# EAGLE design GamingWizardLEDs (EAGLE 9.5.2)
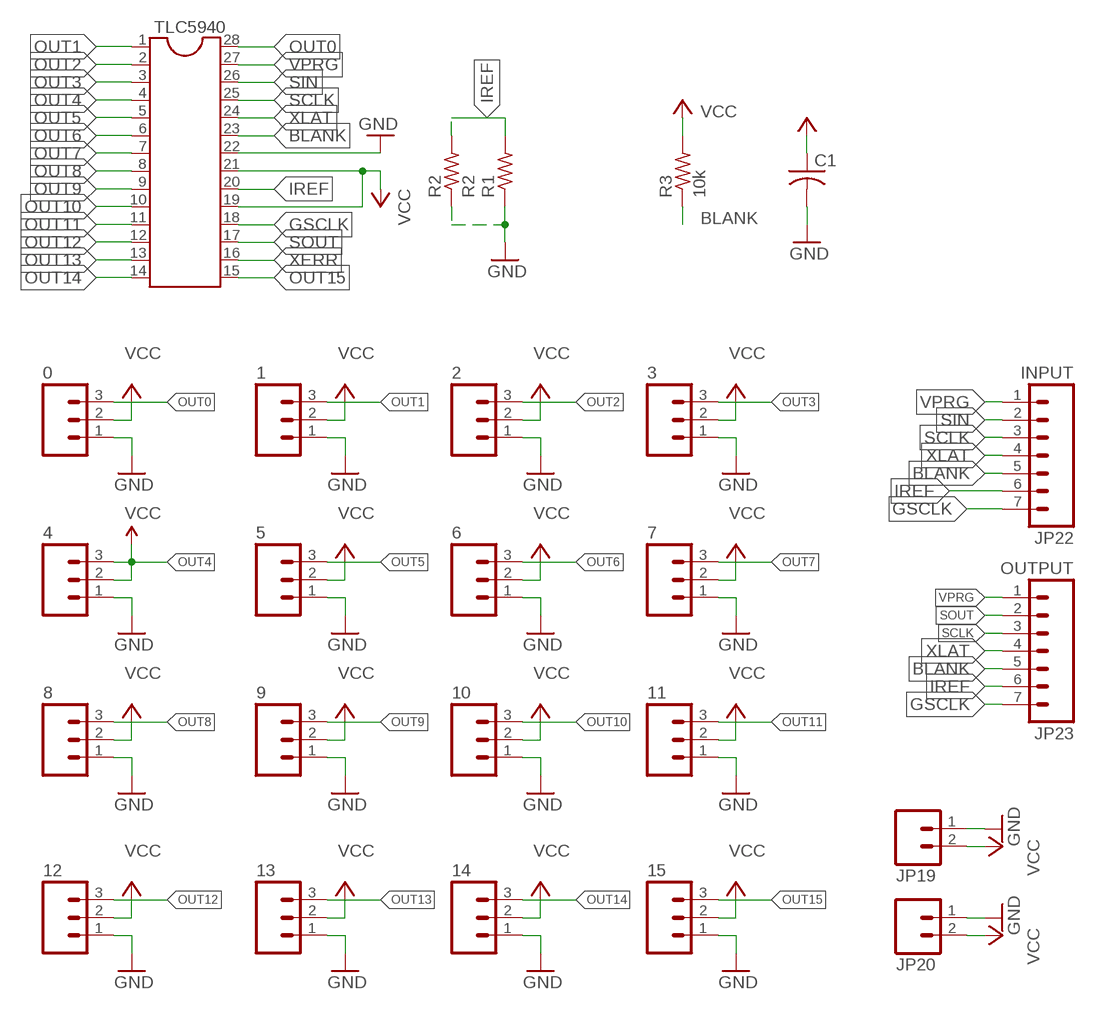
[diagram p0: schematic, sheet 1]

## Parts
0  M03PTH  [1X03]
1  M03PTH  [1X03]
2  M03PTH  [1X03]
3  M03PTH  [1X03]
4  M03PTH  [1X03]
5  M03PTH  [1X03]
6  M03PTH  [1X03]
7  M03PTH  [1X03]
8  M03PTH  [1X03]
9  M03PTH  [1X03]
10  M03PTH  [1X03]
11  M03PTH  [1X03]
12  M03PTH  [1X03]
13  M03PTH  [1X03]
14  M03PTH  [1X03]
15  M03PTH  [1X03]
C1  100nF  C-USC0805  [C0805]
JP19  M02PTH  [1X02]
JP20  M02PTH  [1X02]
JP22  INPUT  M07  [1X07]
JP23  OUTPUT  M07  [1X07]
R1  2.2k  R-US_R0805  [R0805]
R2  R2  R-US_R0805  [R0805]
R3  10k  R-US_R0805  [R0805]
TLC5940  DIL28-3  [DIL28-3]

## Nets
BLANK: JP22.5 JP23.5 R3.1 TLC5940.23
GND: 0.1 1.1 2.1 3.1 4.1 5.1 6.1 7.1 8.1 9.1 10.1 11.1 12.1 13.1 14.1 15.1 C1.2 JP19.1 JP20.1 R1.1 R2.1 TLC5940.22
GSCLK: JP22.7 JP23.7 TLC5940.18
IREF: JP22.6 JP23.6 R1.2 R2.2 TLC5940.20
OUT0: 0.3 TLC5940.28
OUT1: 1.3 TLC5940.1
OUT2: 2.3 TLC5940.2
OUT3: 3.3 TLC5940.3
OUT4: 4.3 TLC5940.4
OUT5: 5.3 TLC5940.5
OUT6: 6.3 TLC5940.6
OUT7: 7.3 TLC5940.7
OUT8: 8.3 TLC5940.8
OUT9: 9.3 TLC5940.9
OUT10: 10.3 TLC5940.10
OUT11: 11.3 TLC5940.11
OUT12: 12.3 TLC5940.12
OUT13: 13.3 TLC5940.13
OUT14: 14.3 TLC5940.14
OUT15: 15.3 TLC5940.15
SCLK: JP22.3 JP23.3 TLC5940.25
SIN: JP22.2 TLC5940.26
SOUT: JP23.2 TLC5940.17
VCC: 0.2 1.2 2.2 3.2 4.2 5.2 6.2 7.2 8.2 9.2 10.2 11.2 12.2 13.2 14.2 15.2 C1.1 JP19.2 JP20.2 R3.2 TLC5940.19 TLC5940.21
VPRG: JP22.1 JP23.1 TLC5940.27
XERR: TLC5940.16
XLAT: JP22.4 JP23.4 TLC5940.24

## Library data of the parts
0 1-15 = SparkFun:M03: Header 3 Standard 3-pin 0.1" header. Use with straight break away headers (SKU : PRT-00116), right angle break away headers (PRT-00553), swiss pins (PRT-00743), machine pins (PRT-00117), and female headers (PRT-00115). Molex polarized connector foot print use with SKU : PRT-08232 with associated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
C1 = rcl:C-US: CAPACITOR, American symbol; MANUFACTURER: Samsung Electro-Mechanics; MANUFACTURER_PART_NUMBER: CL21F104ZBCNNNC; SPICEPREFIX: C
JP19 JP20 = SparkFun:M02: Header 2
JP22 JP23 = SparkFun:M07: Header 7 Standard 7-pin 0.1" header. Use with straight break away headers (SKU : PRT-00116), right angle break away headers (PRT-00553), swiss pins (PRT-00743), machine pins (PRT-00117), and female headers (PRT-00115). NOTES ON THE VARIANTS LOCK and LOCK_LONGPADS... This footprint was designed to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
R1 = rcl:R-US_: RESISTOR, American symbol; MANUFACTURER: UNI-ROYAL(Uniroyal Elec); MANUFACTURER_PART_NUMBER: 0805W8J0222T5E; SPICEPREFIX: R
R2 = rcl:R-US_: RESISTOR, American symbol; SPICEPREFIX: R
R3 = rcl:R-US_: RESISTOR, American symbol; MANUFACTURER: UNI-ROYAL(Uniroyal Elec); MANUFACTURER_PART_NUMBER: 0805W8F1002T5E; SPICEPREFIX: R
TLC5940 = ic-package:DIL28: Dual In Line

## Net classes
0 default: width 0.508 mm

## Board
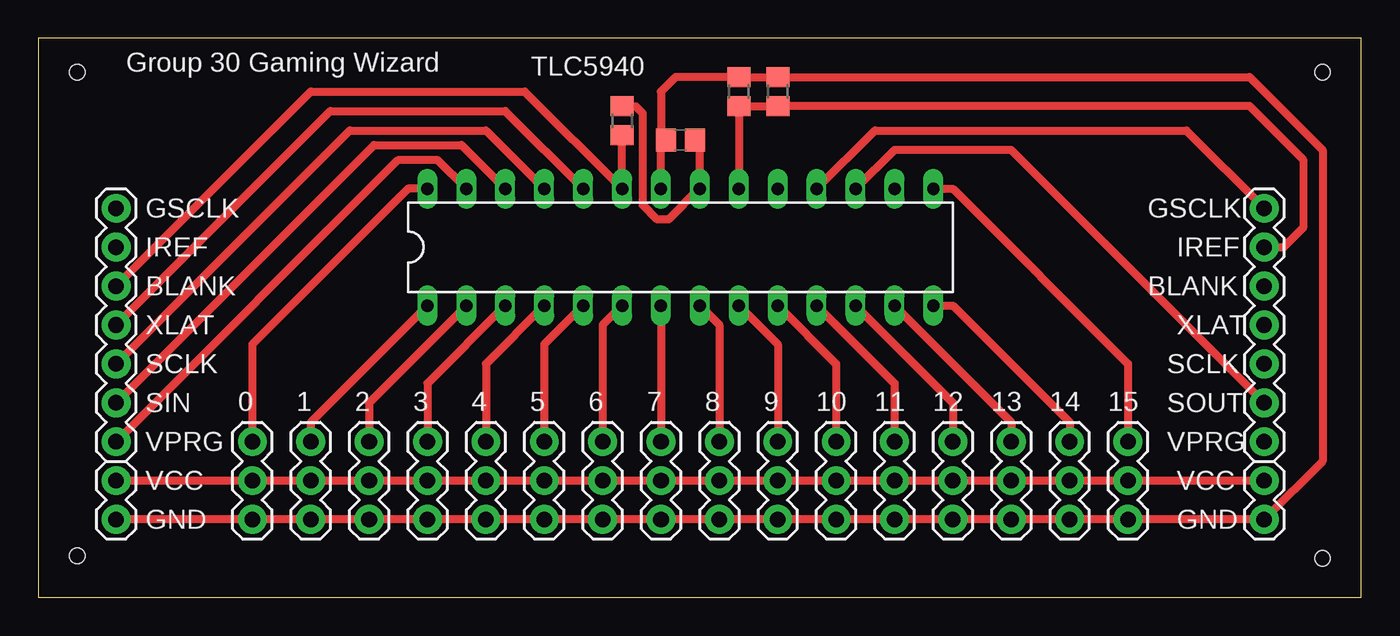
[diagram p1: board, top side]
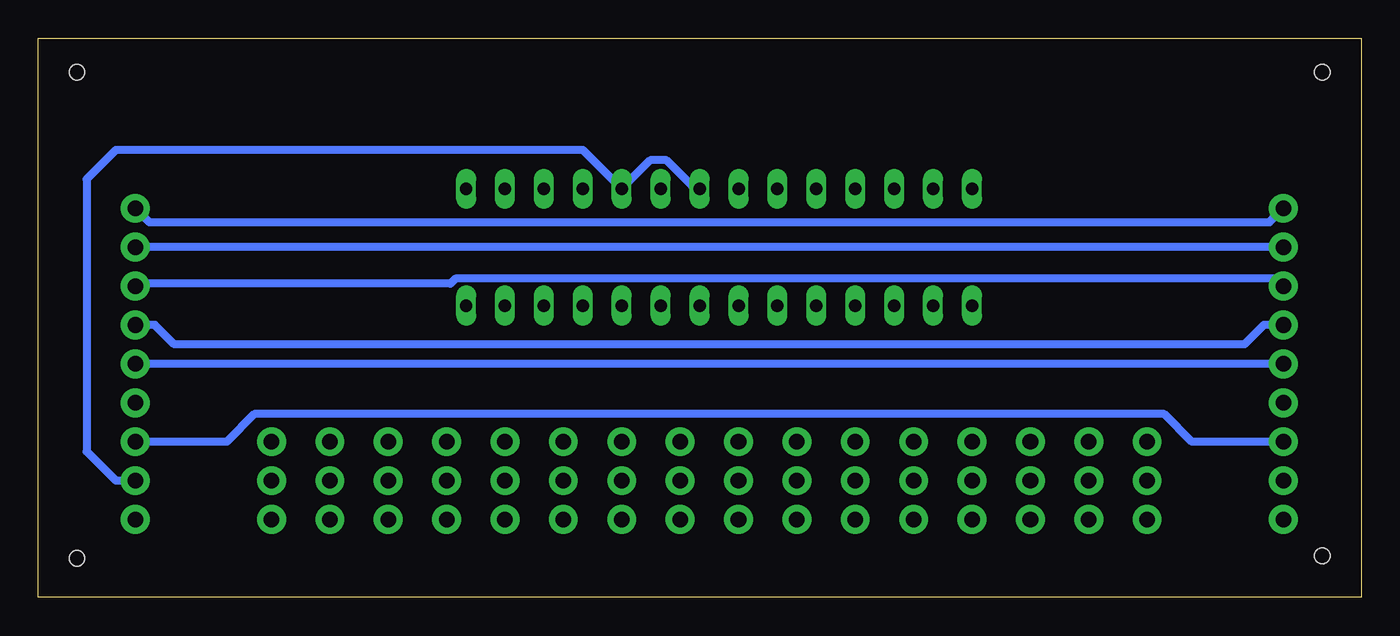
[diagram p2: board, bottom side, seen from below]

Size 86.34 x 36.5 mm. Coordinates in mm from the lower left corner, seen from the top.
Outline: 0,0 86.34,0 86.34,36.5 0,36.5 0,0
Copper layers (1*16): Top 0.035mm / dielectric 1.5mm / Bottom 0.035mm
Design rules "default": minimum track width 6mil, minimum drill 0.35mm, track to track 6mil, track to pad 6mil, pad to pad 6mil, via to via 6mil, smd to smd 6mil, copper to edge 40mil, drill to drill 6mil, minimum pad ring 10mil, minimum via ring 8mil, stop-mask expansion 4mil, vias tented up to drill 0mil, thermal gap 10mil
Holes 1 mm at 2.54,2.7 2.54,34.29 83.82,34.29 83.82,2.54

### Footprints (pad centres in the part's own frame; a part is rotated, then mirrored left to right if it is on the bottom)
1X03 = drill 1.016 pad 1.88: 1 0,0; 2 2.54,0; 3 5.08,0
C0805 = smd 1.3 x 1.5: 1 -0.95,0; 2 0.95,0
1X02 = drill 1.016 pad 1.88: 1 0,0; 2 2.54,0
1X07 = drill 1.016 pad 1.88: 1 0,0; 2 2.54,0; 3 5.08,0; 4 7.62,0; 5 10.16,0; 6 12.7,0; 7 15.24,0
R0805 = smd 1.3 x 1.5: 1 -0.95,0; 2 0.95,0
DIL28-3 = drill 0.813 long: 1 -16.51,-3.81; 2 -13.97,-3.81; 3 -11.43,-3.81; 4 -8.89,-3.81; 5 -6.35,-3.81; 6 -3.81,-3.81; 7 -1.27,-3.81; 8 1.27,-3.81; 9 3.81,-3.81; 10 6.35,-3.81; 11 8.89,-3.81; 12 11.43,-3.81; 13 13.97,-3.81; 14 16.51,-3.81; 15 16.51,3.81; 16 13.97,3.81; 17 11.43,3.81; 18 8.89,3.81; 19 6.35,3.81; 20 3.81,3.81; 21 1.27,3.81; 22 -1.27,3.81; 23 -3.81,3.81; 24 -6.35,3.81; 25 -8.89,3.81; 26 -11.43,3.81; 27 -13.97,3.81; 28 -16.51,3.81

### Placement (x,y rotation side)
0  13.97,5.08 90 top
1  17.78,5.08 90 top
2  21.59,5.08 90 top
3  25.4,5.08 90 top
4  29.21,5.08 90 top
5  33.02,5.08 90 top
6  36.83,5.08 90 top
7  40.64,5.08 90 top
8  44.45,5.08 90 top
9  48.26,5.08 90 top
10  52.07,5.08 90 top
11  55.88,5.08 90 top
12  59.69,5.08 90 top
13  63.5,5.08 90 top
14  67.31,5.08 90 top
15  71.12,5.08 90 top
C1  41.91,29.84 180 top
JP19  5.08,5.08 90 top
JP20  80.01,5.08 90 top
JP22  5.08,10.16 90 top
JP23  80.01,10.16 90 top
R1  45.72,33.02 270 top
R2  48.26,33.02 270 top
R3  38.1,31.11 90 top
TLC5940  41.91,22.86 0 top

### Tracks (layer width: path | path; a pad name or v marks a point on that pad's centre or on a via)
BLANK
  Top 0.508: JP22.5 17.78,33.02 31.75,33.02 TLC5940.23 R3.1
  Bottom 0.508: JP22.5 5.28,20.47 5.61,20.8 59.11,20.8 59.44,20.47 79.91,20.47 JP23.5
GND
  Top 0.508: JP19.1 0.1 1.1 2.1 3.1 4.1 5.1 6.1 7.1 8.1 9.1 10.1 11.1 12.1 13.1 14.1 15.1 JP20.1 83.82,8.89 83.82,29.21 79.06,33.97 R2.1 R1.1 41.59,33.97 40.64,33.02 40.64,29.84 40.8,29.68 | TLC5940.22 40.64,29.52 40.8,29.68 | 40.8,29.68 C1.2
GSCLK
  Top 0.508: TLC5940.18 54.61,30.48 74.93,30.48 JP23.7
  Bottom 0.508: JP22.7 5.99,24.49 79.1,24.49 JP23.7
IREF
  Top 0.508: TLC5940.20 R1.2 R2.2 79.06,32.07 82.55,28.57 82.55,24.13 81.28,22.86 JP23.6
  Bottom 0.508: JP22.6 JP23.6
OUT0
  Top 0.508: TLC5940.28 24.13,26.67 13.97,16.51 0.3
OUT1
  Top 0.508: TLC5940.1 17.78,11.43 1.3
OUT2
  Top 0.508: TLC5940.2 21.59,12.7 2.3
OUT3
  Top 0.508: TLC5940.3 25.4,13.97 3.3
OUT4
  Top 0.508: TLC5940.4 29.21,15.24 4.3
OUT5
  Top 0.508: TLC5940.5 33.02,16.51 5.3
OUT6
  Top 0.508: TLC5940.6 36.83,17.78 6.3
OUT7
  Top 0.508: TLC5940.7 7.3
OUT8
  Top 0.508: TLC5940.8 44.45,17.78 8.3
OUT9
  Top 0.508: TLC5940.9 48.26,16.51 9.3
OUT10
  Top 0.508: TLC5940.10 52.07,15.24 10.3
OUT11
  Top 0.508: TLC5940.11 55.88,13.97 11.3
OUT12
  Top 0.508: TLC5940.12 59.69,12.7 12.3
OUT13
  Top 0.508: TLC5940.13 63.5,11.43 13.3
OUT14
  Top 0.508: TLC5940.14 59.69,19.05 67.31,11.43 14.3
OUT15
  Top 0.508: TLC5940.15 59.69,26.67 71.12,15.24 15.3
SCLK
  Top 0.508: JP22.3 20.32,30.48 29.21,30.48 TLC5940.25
  Bottom 0.508: JP22.3 JP23.3
SIN
  Top 0.508: JP22.2 21.91,29.53 27.62,29.53 TLC5940.26
SOUT
  Top 0.508: JP23.2 63.5,29.21 55.88,29.21 TLC5940.17
VCC
  Top 0.508: JP19.2 0.2 1.2 2.2 3.2 4.2 5.2 6.2 7.2 8.2 9.2 10.2 11.2 12.2 13.2 14.2 15.2 JP20.2 | C1.1 43.18,29.52 TLC5940.21 43.13,26.67 41.13,24.68 40.39,24.68 39.47,25.6 39.47,31.59 38.99,32.06 R3.2
  Bottom 0.508: TLC5940.21 43.48,26.67 45.35,28.54 46.41,28.54 48.26,26.68 TLC5940.19 50.8,29.21 81.28,29.21 83.19,27.3 83.19,9.53 81.28,7.62 JP20.2
VPRG
  Top 0.508: JP22.1 23.46,28.54 26.07,28.54 TLC5940.27
  Bottom 0.508: JP22.1 11.05,10.16 12.85,11.96 72.24,11.96 74.04,10.16 JP23.1
XLAT
  Top 0.508: JP22.4 19.05,31.75 30.48,31.75 TLC5940.24
  Bottom 0.508: JP22.4 6.35,17.78 7.62,16.51 77.47,16.51 78.74,17.78 JP23.4

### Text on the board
tNames: Group 30 Gaming Wizard | GSCLK | GSCLK | IREF | IREF | BLANK | BLANK | XLAT | XLAT | SCLK | SCLK | SIN | SOUT | VPRG | VPRG | VCC | VCC | GND | GND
